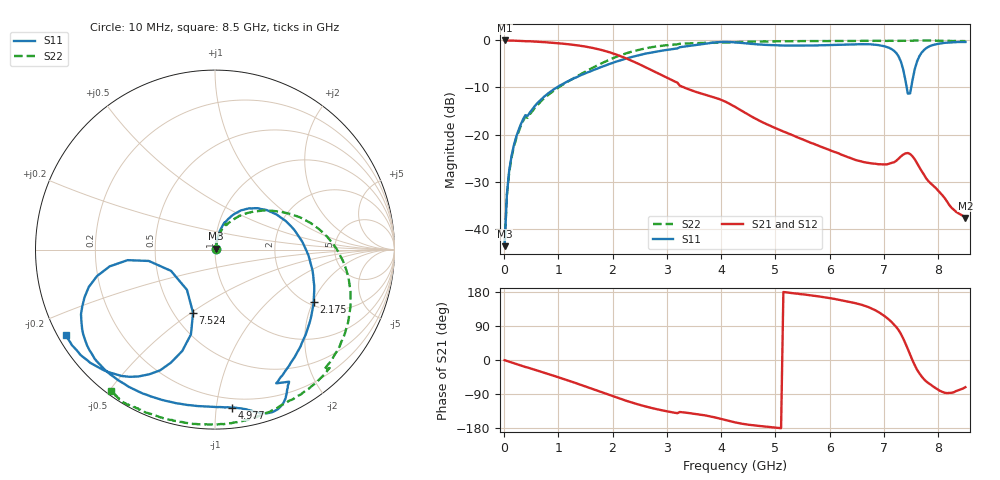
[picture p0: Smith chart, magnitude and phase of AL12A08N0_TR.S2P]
!AVX CORPORATION
!PART NUMBER AL12A08N0_TR
!DESCRIPTION: AIR CORE INDUCTOR, 8nH, 3 TURNS
!Agilent Technologies,E5071C,MY46102230,A.09.54
!Date: Mon Sep 03 15:49:23 2012
!Data & Calibration Information:
!Freq	S11:SOLT2(ON)	S21:SOLT2(ON)	S12:SOLT2(ON)	S22:SOLT2(ON)
# Hz S RI R 50
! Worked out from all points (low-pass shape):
!   201 points, 10 MHz to 8.5 GHz, reference 50 ohm
!   highest |S21| = -0.05 dB at 10 MHz (marker M1); lowest = -37.6 dB at 8.5 GHz (marker M2)
!   |S21| within 3 dB of the highest: start of sweep to 2.071 GHz
!   lowest |S11| = -43.6 dB at 10 MHz (marker M3), VSWR 1.01, Z = 50.5 + j0.455 ohm
!   |S11| at or under -10 dB: start of sweep to 971.2 MHz; 7.419 GHz to 7.501 GHz (82.37 MHz wide, 1.1 % of centre)
!   |S22| runs from -43.4 to -0.1 dB; largest |S21 - S12| = 0.0025
!   S11 on the Smith chart (normalised r, x): 10 MHz: 1.01, +0.01; 2.175 GHz: 2.14, -2.02; 4.977 GHz: 0.13, -1.10; 7.524 GHz: 0.62, -0.51; 8.5 GHz: 0.02, -0.27
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1e7  0.00483 0.0045  0.9946 -0.00892  0.994 -0.00857  0.00507 0.00452
5.245e7  0.00637 0.0227  0.9929 -0.0438  0.9949 -0.0435  0.00652 0.0221
9.49e7  0.00866 0.0408  0.9893 -0.0787  0.9896 -0.0788  0.00966 0.0388
1.798e8  0.0168 0.0752  0.9785 -0.1469  0.9797 -0.1468  0.0189 0.0719
3.496e8  0.0449 0.138  0.94 -0.2771  0.9414 -0.2784  0.05 0.1302
9.8635e8  0.2223 0.2308  0.6585 -0.6567  0.6589 -0.6576  0.2276 0.2138
1.4533e9  0.4109 0.1429  0.3313 -0.7994  0.3306 -0.7998  0.402 0.2029
2.17495e9  0.5496 -0.2899  -0.1619 -0.6489  -0.1618 -0.6486  0.7017 -0.0406
2.85415e9  0.4136 -0.6458  -0.2893 -0.3316  -0.2897 -0.3315  0.7161 -0.4885
3.19375e9  0.3411 -0.7451  -0.2738 -0.227  -0.274 -0.2269  0.6077 -0.6696
4.255e9  0.2661 -0.9112  -0.1904 -0.0526  -0.1903 -0.0524  0.2874 -0.9089
4.97665e9  0.0927 -0.8809  -0.119 -0.00453  -0.1189 -0.00438  0.033 -0.9716
5.6983e9  -0.1733 -0.8624  -0.0791 0.0145  -0.079 0.0145  -0.1818 -0.9608
6.58975e9  -0.5981 -0.6834  -0.043 0.0293  -0.0427 0.0292  -0.3633 -0.9155
7.09915e9  -0.7466 -0.36  -0.0134 0.0475  -0.0136 0.0476  -0.4389 -0.8838
7.2265e9  -0.7029 -0.2078  0.00285 0.0529  0.003 0.0529  -0.4519 -0.8771
7.35385e9  -0.4867 -0.0588  0.0337 0.0516  0.0339 0.0514  -0.4641 -0.871
7.43875e9  -0.2452 -0.1184  0.0559 0.0312  0.0559 0.031  -0.472 -0.8686
7.52365e9  -0.1221 -0.3524  0.0592 -0.000327  0.0592 -0.00025  -0.4836 -0.863
7.651e9  -0.2463 -0.6303  0.0374 -0.0261  0.0369 -0.026  -0.4996 -0.8554
7.77835e9  -0.4263 -0.7068  0.019 -0.0287  0.019 -0.0287  -0.5135 -0.846
8.5e9  -0.8304 -0.4784  0.00412 -0.0125  0.00412 -0.0126  -0.5816 -0.7864
